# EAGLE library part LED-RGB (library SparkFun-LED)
LED-RGB 6 pin RGB LED (no common connector) Packages: PLCC-6 LED-TRICOLOR-5050 - No built-in IC SparkFun Products: Digital Sandbox LED- SMD RGB
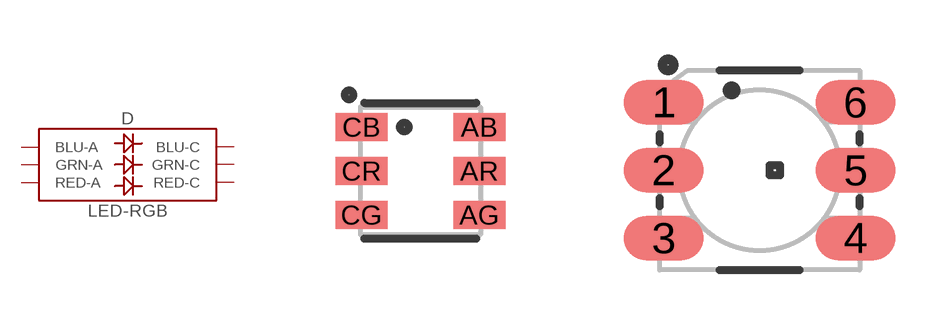
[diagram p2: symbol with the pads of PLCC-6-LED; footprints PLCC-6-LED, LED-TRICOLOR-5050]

Designator prefix D

## LED-RGBPLCC-6 (PROD_ID: DIO-12113; VALUE: RGB)  [PLCC-6-LED]
AB  BLU-A
AG  GRN-A
AR  RED-A
CB  BLU-C
CG  GRN-C
CR  RED-C

## LED-RGBNO_IC (PROD_ID: DIO-10298)  [LED-TRICOLOR-5050]
1  GRN-A
2  RED-A
3  BLU-A
4  BLU-C
5  RED-C
6  GRN-C

## Footprint PLCC-6-LED (pad centres in mm)
PLCC-6-LED Specifications: Pin count: 6 Size: 3.2*2.8*1.39mm Datasheet referenced for footprint: LTRB GFSF Example device: RGB-LED-PLCC
smd 1.3 x 0.7: AB 1.475,1.1; AG 1.475,-1.1; AR 1.475,0; CB -1.475,1.1; CG -1.475,-1.1; CR -1.475,0

## Footprint LED-TRICOLOR-5050 (pad centres in mm)
5050 SMD RGB LED Specifications: Pin count: 6 Pin pitch: 0.6mm Area: 5.0mm x 5.mm Thickness: 2.6mm Datasheet referenced for footprint: 5060BRG4 Example device(s): LED-RGB
smd 2 x 1.1: 1 -2.4,1.7; 2 -2.4,0; 3 -2.4,-1.7; 4 2.4,-1.7; 5 2.4,0; 6 2.4,1.7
